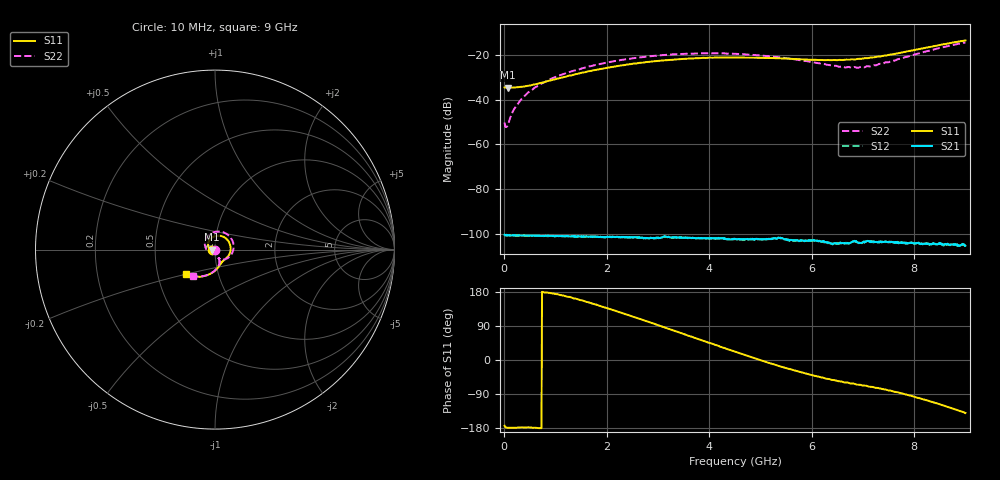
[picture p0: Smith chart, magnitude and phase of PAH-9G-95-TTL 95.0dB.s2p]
! MTS Systemtechnik GmbH
! S-Parameters
! Model: PAH-9G/95-TTL
! Attenuation Step: 95.0dB
#  HZ  S  DB  R  50.00
! Rohde & Schwarz Vector Network Analyzer
! Rohde-Schwarz,ZNB20-2Port,1334333062101652,3.45
! Created: UTC 1/26/2024, 8:22:13 AM
! freq[Hz]  db:S11  ang:S11  db:S21  ang:S21  db:S12  ang:S12  db:S22  ang:S22
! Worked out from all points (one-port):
!   900 points, 10 MHz to 9 GHz, reference 50 ohm
!   lowest |S11| = -34.6 dB at 80 MHz (marker M1), VSWR 1.04, Z = 48.2 - j0.0352 ohm
!   |S11| at or under -10 dB: start of sweep to end of sweep
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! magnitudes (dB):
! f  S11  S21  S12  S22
! 10 MHz  -34.4  -100.4  -100.5  -50.2
! 50 MHz  -34.5  -100.5  -100.4  -52.1
! 80 MHz  -34.6  -100.6  -100.6  -50.9
! 160 MHz  -34.6  -100.6  -100.6  -45.7
! 220 MHz  -34.5  -100.8  -100.7  -43.3
! 330 MHz  -34.2  -100.7  -100.8  -39.8
! 480 MHz  -33.7  -100.7  -100.9  -36.5
! 720 MHz  -32.5  -101.0  -100.8  -32.8
! 910 MHz  -31.3  -100.8  -101.0  -30.7
! 1.51 GHz  -27.9  -101.4  -101.2  -26.0
! 2.14 GHz  -25.2  -101.4  -101.4  -22.7
! 3.01 GHz  -22.6  -101.9  -102.0  -20.1
! 3.78 GHz  -21.4  -102.0  -101.9  -19.2
! 4.51 GHz  -21.1  -102.2  -102.3  -19.4
! 5.2 GHz  -21.3  -102.3  -102.3  -20.5
! 6.01 GHz  -22.1  -102.9  -103.1  -23.1
! 6.53 GHz  -22.1  -104.3  -104.3  -25.2
! 6.79 GHz  -21.9  -103.6  -103.7  -25.7
! 7.14 GHz  -21.1  -103.6  -103.7  -25.1
! 7.51 GHz  -19.8  -103.8  -103.5  -23.1
! 8.47 GHz  -15.6  -104.5  -104.9  -16.9
! 9 GHz  -13.4  -105.3  -105.5  -14.3
